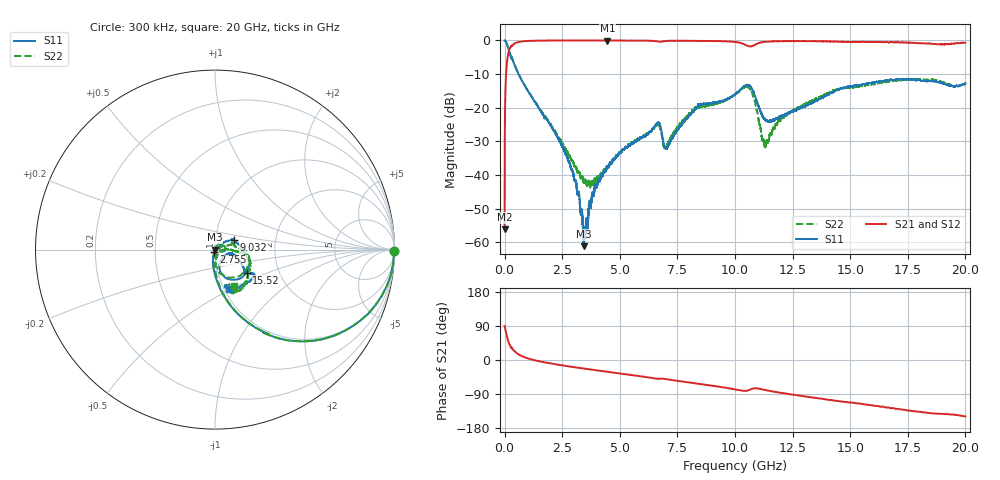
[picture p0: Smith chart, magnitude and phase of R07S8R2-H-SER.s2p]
!{R07S8R2}
!Johanson Technology Inc.
!www.johansontechnology.com
!Test Board Conditions:
!Substrate Type  RO4350B
!Substrate Thickness  10 mil
!Substrate Dk  3.66
!TL Type: GCPW
!TL Trace Width  21 mil
!TL Gap  20 mil
!Electrode orientation  Horizontal
!DUT TOPOLOGY	SERIES
!Mounting Pad LxW  16x21 mil
! Created Sat Feb  6 11:40:28 2021
# hz S ma R 50
! 2 Port Network Data from SP1.SP block
! freq  magS11  angS11  magS21  angS21  magS12  angS12  magS22  angS22
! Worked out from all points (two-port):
!   20001 points, 300 kHz to 20 GHz, reference 50 ohm
!   highest |S21| = -0.02 dB at 4.463 GHz (marker M1); lowest = -56.2 dB at 300 kHz (marker M2)
!   |S21| within 3 dB of the highest: 193.1 MHz to end of sweep
!   lowest |S11| = -61.2 dB at 3.443 GHz (marker M3), VSWR 1.00, Z = 49.9 + j0.00726 ohm
!   |S11| at or under -10 dB: 608 MHz to end of sweep
!   |S22| runs from -43.8 to 0.0 dB; largest |S21 - S12| = 0.013
!   S11 on the Smith chart (normalised r, x): 300 kHz: open; 2.755 GHz: 0.99, -0.03; 9.032 GHz: 1.23, +0.13; 15.52 GHz: 1.37, -0.37; 20 GHz: 1.05, -0.48
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300000  0.9984 -0.5  0.001558 89.7  0.001561 91.0  0.9984 -0.4
1.083e8  0.8692 -30.2  0.4894 60.2  0.49 60.1  0.8696 -30.0
2.623e8  0.5861 -56.0  0.8037 34.6  0.8031 34.6  0.5878 -56.0
8.413e8  0.2229 -82.3  0.9741 8.0  0.9733 8.0  0.2242 -81.5
2.7553e9  0.01647 -114.2  0.9963 -16.5  0.9964 -16.5  0.02062 -81.5
3.1553e9  0.00551 -128.4  0.9961 -20.1  0.9966 -20.1  0.01126 -59.4
3.3343e9  0.002867 -142.6  0.9963 -21.6  0.9968 -21.6  0.009093 -49.1
3.4433e9  0.0008712 175.2  0.9961 -22.6  0.9971 -22.5  0.007585 -34.9
3.8733e9  0.005168 61.2  0.9969 -26.2  0.9966 -26.2  0.007637 9.8
4.4633e9  0.01345 43.3  0.9979 -31.1  0.9965 -31.1  0.01339 54.3
6.6673e9  0.06002 8.2  0.9634 -49.6  0.9631 -49.6  0.05718 14.1
7.0293e9  0.02473 16.6  0.9825 -50.7  0.984 -50.6  0.02601 16.4
8.2863e9  0.09561 32.2  0.9852 -61.7  0.9859 -61.7  0.1008 18.0
9.0323e9  0.1187 26.8  0.9809 -68.0  0.9807 -68.1  0.1122 11.2
1.00003e10  0.1584 1.2  0.9502 -77.5  0.9511 -77.6  0.1556 -2.3
1.06633e10  0.2084 -52.6  0.814 -77.9  0.8146 -77.9  0.1867 -55.4
1.13493e10  0.06483 -54.9  0.9587 -79.5  0.9583 -79.6  0.02958 -35.9
1.19723e10  0.0721 -21.7  0.9762 -86.4  0.9758 -86.4  0.06403 1.8
1.33343e10  0.1178 -16.5  0.9753 -98.7  0.976 -98.7  0.1261 -5.9
1.55163e10  0.219 -35.8  0.9568 -116.2  0.9545 -116.1  0.2107 -22.0
1.66673e10  0.2515 -32.1  0.9367 -125.4  0.9419 -125.9  0.2452 -43.8
2e10  0.2296 -70.9  0.9267 -149.0  0.9226 -149.0  0.2282 -62.7
